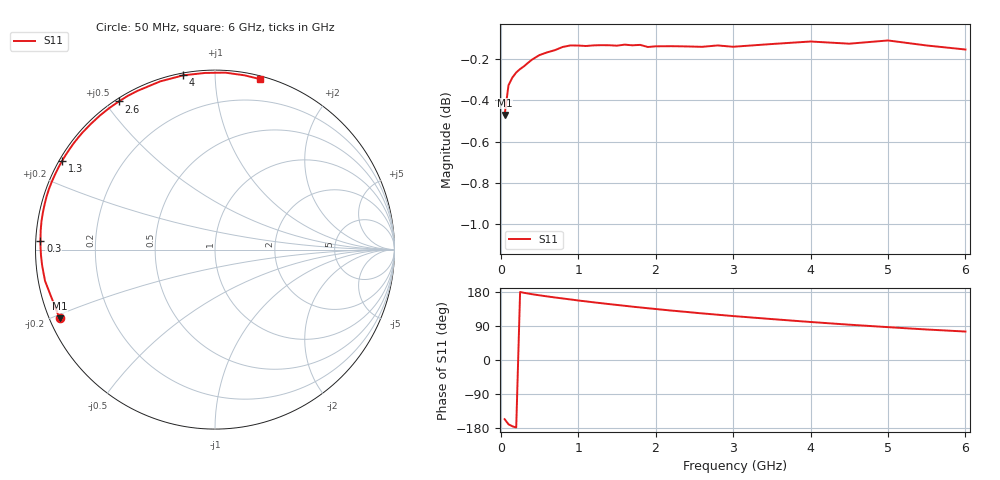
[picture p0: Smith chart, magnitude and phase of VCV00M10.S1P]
! Infineon Technologies  Discrete & RF Semiconductors
! BBY 56-03
! Si Tuning Diode in SOD323
! VR =
! S-Parameters:  June  1999
# GHz  S  MA  R  50
!  f  S11
! GHz  MAG  ANG
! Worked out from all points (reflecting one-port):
!   34 points, 50 MHz to 6 GHz, reference 50 ohm
!   lowest |S11| = -0.5 dB at 50 MHz (marker M1), VSWR 36.88, Z = 1.42 - j10.6 ohm
!   phase of S11 starts at -156 deg and turns -129 deg over the sweep
!   S11 on the Smith chart (normalised r, x): 50 MHz: 0.03, -0.21; 300 MHz: 0.01, +0.02; 1.3 GHz: 0.01, +0.27; 2.6 GHz: 0.01, +0.54; 4 GHz: 0.01, +0.83; 6 GHz: 0.02, +1.30
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0.05  0.9472 -156.1
0.1  0.9631 -169.6
0.15  0.9673 -174.9
0.2  0.9701 -178.2
0.25  0.9719 179.4
0.3  0.9734 177.3
0.4  0.977 173.8
0.5  0.9795 170.7
0.7  0.9822 165.0
0.8  0.984 162.4
1  0.9848 157.1
1.2  0.9849 152.2
1.3  0.985 149.9
1.4  0.9849 147.5
1.6  0.9853 143.1
1.8  0.9851 138.7
2  0.9843 134.6
2.2  0.9844 130.5
2.4  0.9843 126.8
2.6  0.9841 123.0
2.8  0.9848 119.5
3  0.9841 116.0
3.5  0.9856 108.0
4  0.987 100.3
4.5  0.9858 93.2
5  0.9876 86.7
5.5  0.9848 80.5
6  0.9826 75.1
